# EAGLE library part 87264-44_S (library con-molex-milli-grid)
RECEPTACAL
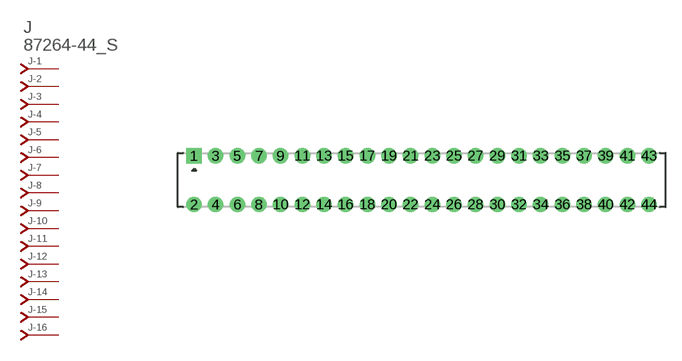
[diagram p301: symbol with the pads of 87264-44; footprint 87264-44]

Designator prefix J; gates -1=J-NV -2=J-N -3=J-N -4=J-N -5=J-N -6=J-N -7=J-N -8=J-N -9=J-N -10=J-N -11=J-N -12=J-N -13=J-N -14=J-N -15=J-N -16=J-N -17=J-N -18=J-N -19=J-N -20=J-N -21=J-N -22=J-N -23=J-N -24=J-N -25=J-N -26=J-N -27=J-N -28=J-N -29=J-N -30=J-N -31=J-N -32=J-N -33=J-N -34=J-N -35=J-N -36=J-N -37=J-N -38=J-N -39=J-N -40=J-N -41=J-N -42=J-N -43=J-N -44=J-N

## 87264-44_S  [87264-44]
1  -1:J  pas
2  -2:J  pas
3  -3:J  pas
4  -4:J  pas
5  -5:J  pas
6  -6:J  pas
7  -7:J  pas
8  -8:J  pas
9  -9:J  pas
10  -10:J  pas
11  -11:J  pas
12  -12:J  pas
13  -13:J  pas
14  -14:J  pas
15  -15:J  pas
16  -16:J  pas
17  -17:J  pas
18  -18:J  pas
19  -19:J  pas
20  -20:J  pas
21  -21:J  pas
22  -22:J  pas
23  -23:J  pas
24  -24:J  pas
25  -25:J  pas
26  -26:J  pas
27  -27:J  pas
28  -28:J  pas
29  -29:J  pas
30  -30:J  pas
31  -31:J  pas
32  -32:J  pas
33  -33:J  pas
34  -34:J  pas
35  -35:J  pas
36  -36:J  pas
37  -37:J  pas
38  -38:J  pas
39  -39:J  pas
40  -40:J  pas
41  -41:J  pas
42  -42:J  pas
43  -43:J  pas
44  -44:J  pas

## Footprint 87264-44 (pad centres in mm)
RECEPTACAL Dual Row, Side Entry
drill 0.914 square: 1 -21,2.25
drill 0.914: 2 -21,-2.25; 3 -19,2.25; 4 -19,-2.25; 5 -17,2.25; 6 -17,-2.25; 7 -15,2.25; 8 -15,-2.25; 9 -13,2.25; 10 -13,-2.25; 11 -11,2.25; 12 -11,-2.25; 13 -9,2.25; 14 -9,-2.25; 15 -7,2.25; 16 -7,-2.25; 17 -5,2.25; 18 -5,-2.25; 19 -3,2.25; 20 -3,-2.25; 21 -1,2.25; 22 -1,-2.25; 23 1,2.25; 24 1,-2.25; 25 3,2.25; 26 3,-2.25; 27 5,2.25; 28 5,-2.25; 29 7,2.25; 30 7,-2.25; 31 9,2.25; 32 9,-2.25; 33 11,2.25; 34 11,-2.25; 35 13,2.25; 36 13,-2.25; 37 15,2.25; 38 15,-2.25; 39 17,2.25; 40 17,-2.25; 41 19,2.25; 42 19,-2.25; 43 21,2.25; 44 21,-2.25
